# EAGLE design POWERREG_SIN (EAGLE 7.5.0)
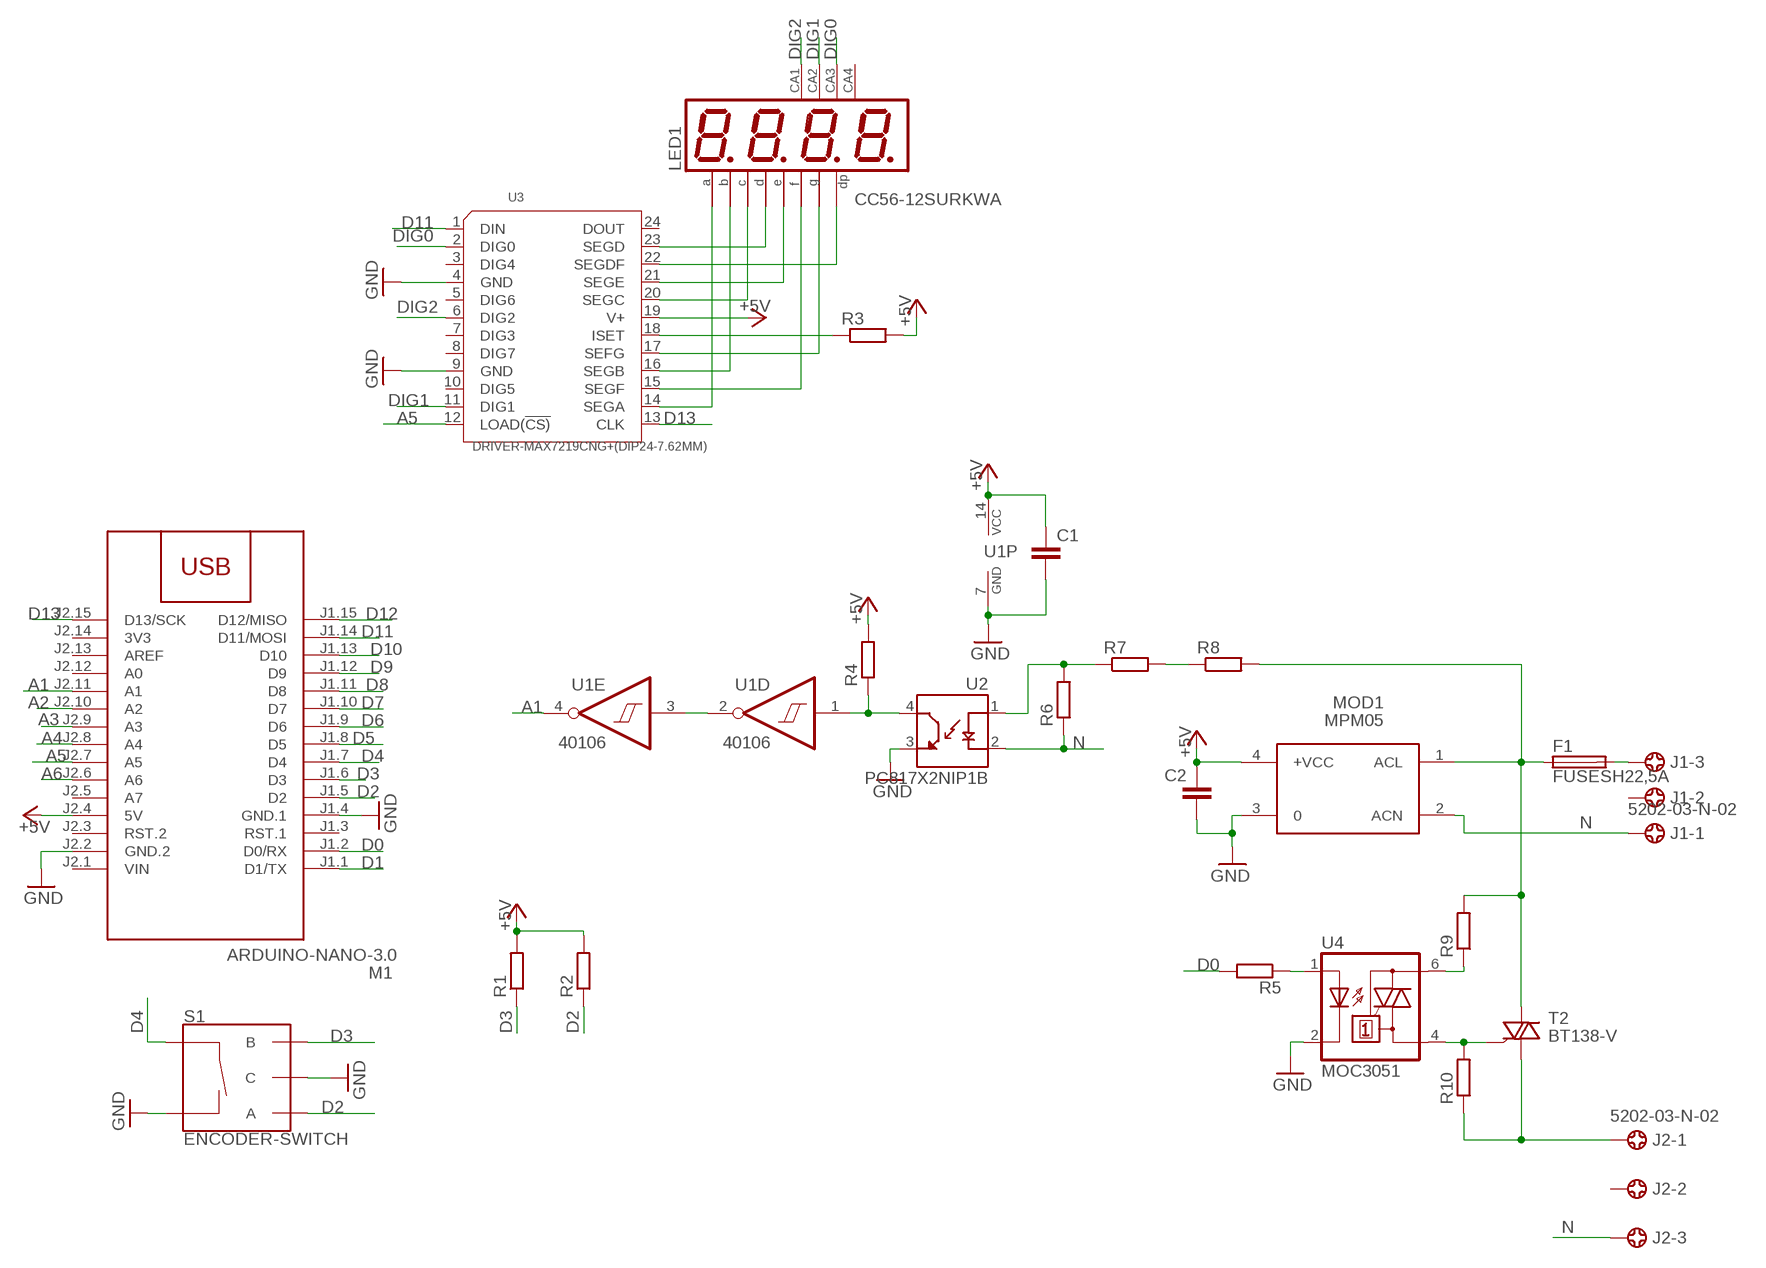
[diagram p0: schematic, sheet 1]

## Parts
C1  C-EUC1206  [C1206]
C2  C-EUC1206  [C1206]
F1  FUSESH22,5A  [SH22,5A]
J1  5202-03-N-02  [5202-03-N-02]
J2  5202-03-N-02  [5202-03-N-02]
LED1  CC56-12SURKWA  CA56-12SURKWA  [CA56-12SURKWA]
M1  ARDUINO-NANO-3.0  [ARDUINO-NANO-3.0]
MOD1  MPM05  [MPM05]
R1  R-EU_R1206  [R1206]
R2  R-EU_R1206  [R1206]
R3  R-EU_R1206  [R1206]
R4  R-EU_R1206  [R1206]
R5  R-EU_R1206  [R1206]
R6  R-EU_R2512  [R2512]
R7  R-EU_R2512  [R2512]
R8  R-EU_R2512  [R2512]
R9  R-EU_R1206  [R1206]
R10  R-EU_R1206  [R1206]
S1  ENCODER-SWITCH  [ROTARY_ENC_PLAIN]
T2  BT138-V  [TO220BV]
U1  40106  74HC14N  [DIL14]
U2  PC817X2NIP1B  [SOIC254P960X420-4N]
U3  DRIVER-MAX7219CNG+(DIP24-7.62MM)  [DIP24-2.54-30.6X7.62MM]
U4  MOC3051  MOC3042M  [DIL06]

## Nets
+5V: C1.1 C2.1 M1.J2.4(5V) MOD1.4(+VCC) R1.2 R2.2 R3.2 R4.2 U1.14(P:VCC) U3.19(V+)
A1: M1.J2.11(A1) U1.4(E:O)
A2: M1.J2.10(A2)
A3: M1.J2.9(A3)
A4: M1.J2.8(A4)
A5: M1.J2.7(A5) U3.12(LOAD(!CS))
A6: M1.J2.6(A6)
D0: M1.J1.2(D0/RX) R5.2
D1: M1.J1.1(D1/TX)
D2: M1.J1.5(D2) R2.1 S1.A
D3: M1.J1.6(D3) R1.1 S1.B
D4: M1.J1.7(D4) S1.SW+
D5: M1.J1.8(D5)
D6: M1.J1.9(D6)
D7: M1.J1.10(D7)
D8: M1.J1.11(D8)
D9: M1.J1.12(D9)
D10: M1.J1.13(D10)
D11: M1.J1.14(D11/MOSI) U3.1(DIN)
D12: M1.J1.15(D12/MISO)
D13: M1.J2.15(D13/SCK) U3.13(CLK)
DIG0: LED1.8(CA) U3.2(DIG0)
DIG1: LED1.9(CA) U3.11(DIG1)
DIG2: LED1.12(CA) U3.6(DIG2)
GND: C1.2 C2.2 M1.J1.4(GND.1) M1.J2.2(GND.2) MOD1.3 S1.C S1.SW- U1.7(P:GND) U2.3(ET) U3.4(GND) U3.9(GND) U4.2(C)
N: J1.1 J2.3 MOD1.2(ACN) R6.1 U2.2(C)
N$1: LED1.11(A) U3.14(SEGA)
N$2: LED1.10(F) U3.15(SEGF)
N$3: LED1.7(B) U3.16(SEGB)
N$4: LED1.5(G) U3.17(SEFG)
N$5: LED1.4(C) U3.20(SEGC)
N$6: LED1.2(D) U3.23(SEGD)
N$7: LED1.1(E) U3.21(SEGE)
N$8: LED1.3(DP) U3.22(SEGDF)
N$9: R3.1 U3.18(ISET)
N$10: F1.2 J1.3
N$11: F1.1 MOD1.1(ACL) R8.2 R9.2 T2.T2(A2)
N$12: R9.1 U4.6(A2)
N$13: R10.2 T2.G U4.4(A1)
N$14: J2.1 R10.1 T2.T1(A1)
N$15: R6.2 R7.1 U2.1(A)
N$16: R7.2 R8.1
N$17: R4.1 U1.1(D:I) U2.4(CT)
N$18: U1.2(D:O) U1.3(E:I)
N$19: R5.1 U4.1(A)
Unconnected: J1.2 J2.2 LED1.6(CA4) M1.J1.3(RST.1) M1.J2.3(RST.2) M1.J2.5(A7) M1.J2.12(A0) M1.J2.13(AREF) U1.5(F:I) U1.6(F:O) U1.8(C:O) U1.9(C:I) U1.10(B:O) U1.11(B:I) U1.12(A:O) U1.13(A:I) U3.3(DIG4) U3.5(DIG6) U3.7(DIG3) U3.8(DIG7) U3.10(DIG5) U3.24(DOUT)

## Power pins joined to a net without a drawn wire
3V3: M1.J2.14(3V3)
VIN: M1.J2.1(VIN)

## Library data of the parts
C1 C2 = rcl:C-EU: CAPACITOR, European symbol
F1 = fuse:FUSE: Fuse; OC_FARNELL: unknown; OC_NEWARK: unknown
J1 J2 = con-ebyelectro:5202-03-N-02: Barrier Blocks Sreies 5202 Source: http://www.ebyelectro.com/PDF/5202-XX-N-02.pdf; OC_FARNELL: unknown; OC_NEWARK: unknown
LED1 = display-kingbright:CA56-12SURKWA
M1 = diy-modules:ARDUINO-NANO-3.0: Arduino Nano 3.0 and compatible devices More details available here: https://www.arduino.cc/en/Main/ArduinoBoardNano Click here to find device on ebay.com
MOD1 = acdc:MPM05: AC DC Converter 5W
R1-R10 = rcl:R-EU_: RESISTOR, European symbol
S1 = SparkFun-Switches:ENCODER-SWITCH: Rotary Encoder w/ Select Switch Encoders rotate similarly to potentiometers, but they’re different from potentiometers in that an encoder has full rotation without limits. They output gray code so that you can tell how much and in which direction the encoder has been turned. This encoder includes a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; SF_SKU: COM-09117
T2 = triac:BT138: TRIAC Source: http://www.semiconductors.philips.com BT138_SERIES_2.pdf
U1 = 74xx-eu:74*14: Hex schmitt trigger INVERTER
U2 = PC817X2NIP1B:PC817X2NIP1B: Check availability; AVAILABILITY: In Stock; CHECK_PRICES: https://www.snapeda.com/parts/PC817X2NIP1B/Sharp/view-part/?ref=eda; DESCRIPTION: Optocoupler DC-IN 1-CH Transistor DC-OUT 4-Pin DIP SMD T/R; MF: Sharp Microelectronics; MP: PC817X2NIP1B; PACKAGE: SMD-4 Sharp Microelectronics; PRICE: None; SNAPEDA_LINK: https://www.snapeda.com/parts/PC817X2NIP1B/Sharp/view-part/?ref=snap
U3 = DRIVER-MAX7219CNG__DIP24-7.62MM_:DRIVER-MAX7219CNG+(DIP24-7.62MM): Check availability; AVAILABILITY: In Stock; CHECK_PRICES: https://www.snapeda.com/parts/MAX7219CNG+/Maxim+Integrated/view-part/?ref=eda; DESCRIPTION: LED Driver 64 Segment 330000uA Supply Current 24-Pin PDIP N Tube; MF: Maxim Integrated Products; MP: MAX7219CNG+; PACKAGE: PDIP-24 Maxim; PRICE: None; SNAPEDA_LINK: https://www.snapeda.com/parts/MAX7219CNG+/Maxim+Integrated/view-part/?ref=snap
U4 = optocoupler:MOC30*: 6-Pin DIP Zero-Cross Optoisolators Triac Driver Output (250/400 Volt Peak) Source: The old path of data sheet not more available 2013-05-06.; MF: FAIRCHILD SEMICONDUCTOR; MPN: MOC3042-M; OC_FARNELL: 1021368; OC_NEWARK: 72K8899

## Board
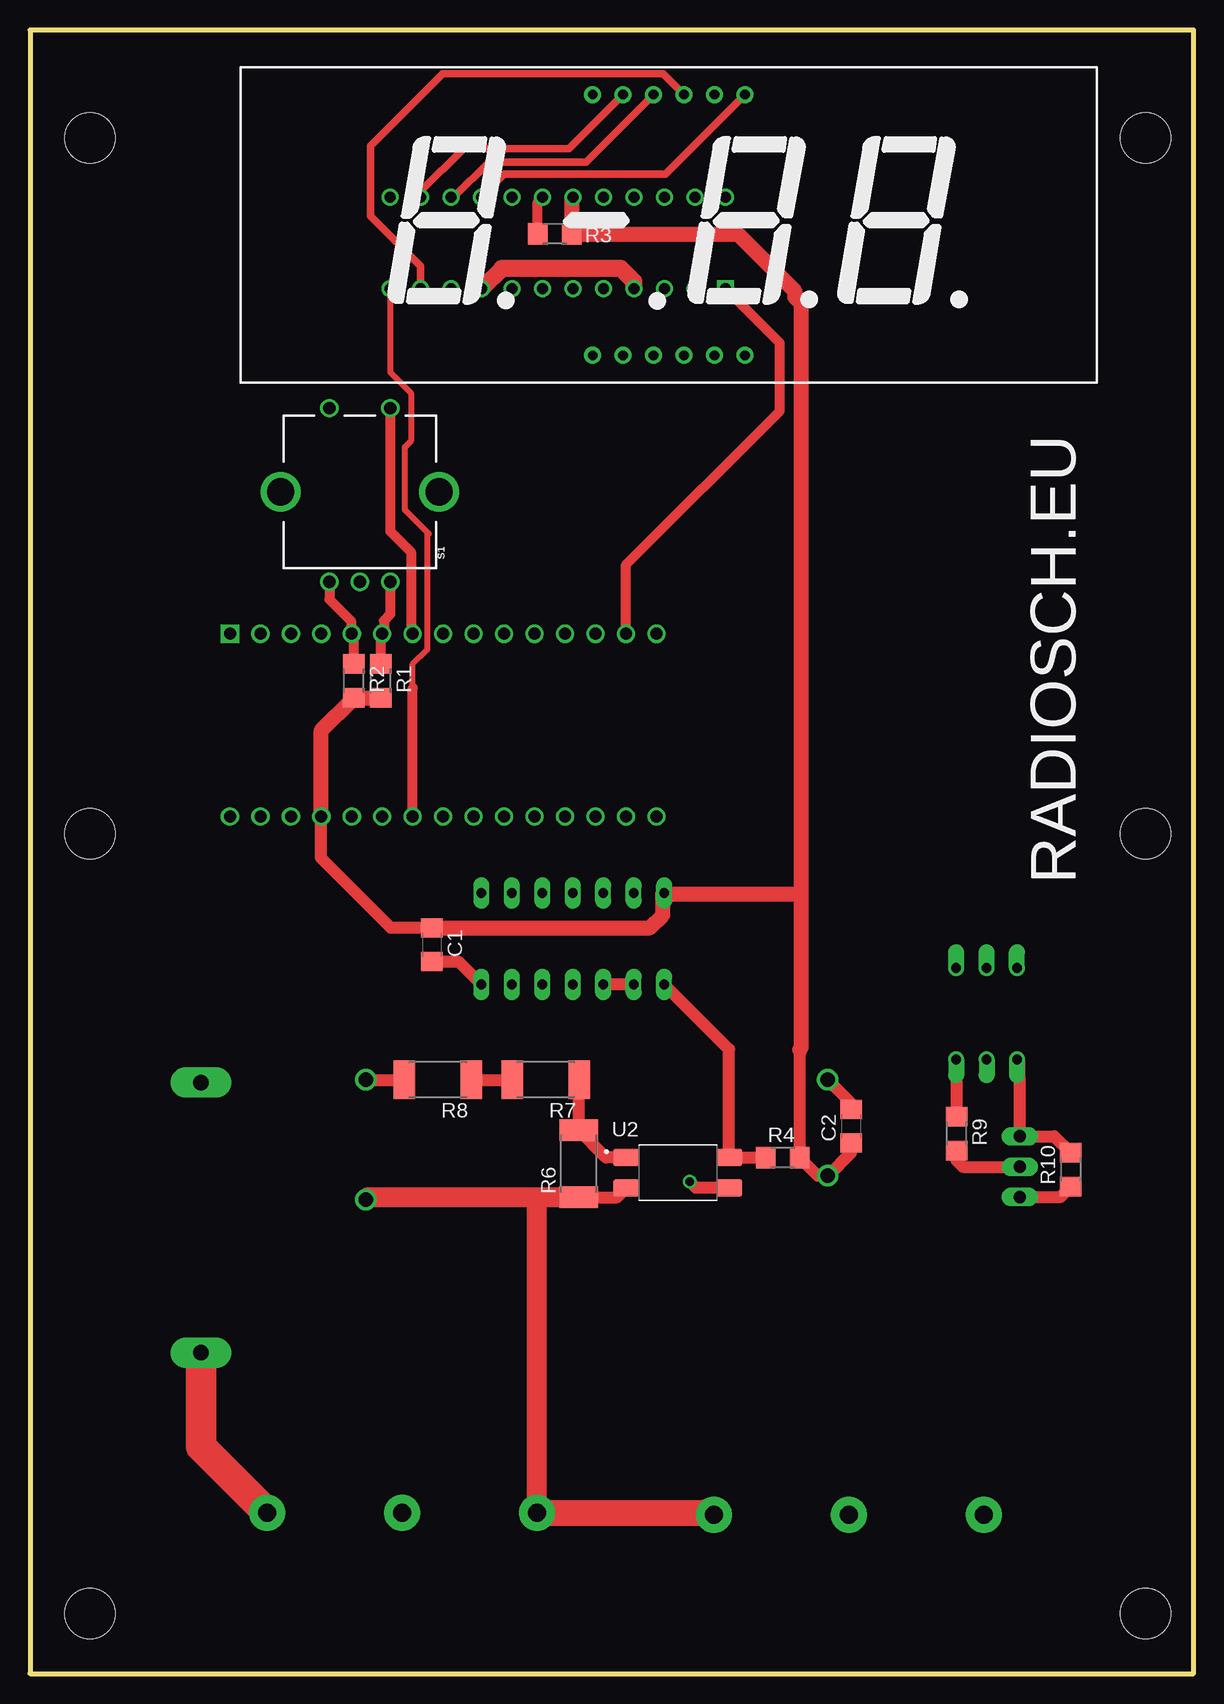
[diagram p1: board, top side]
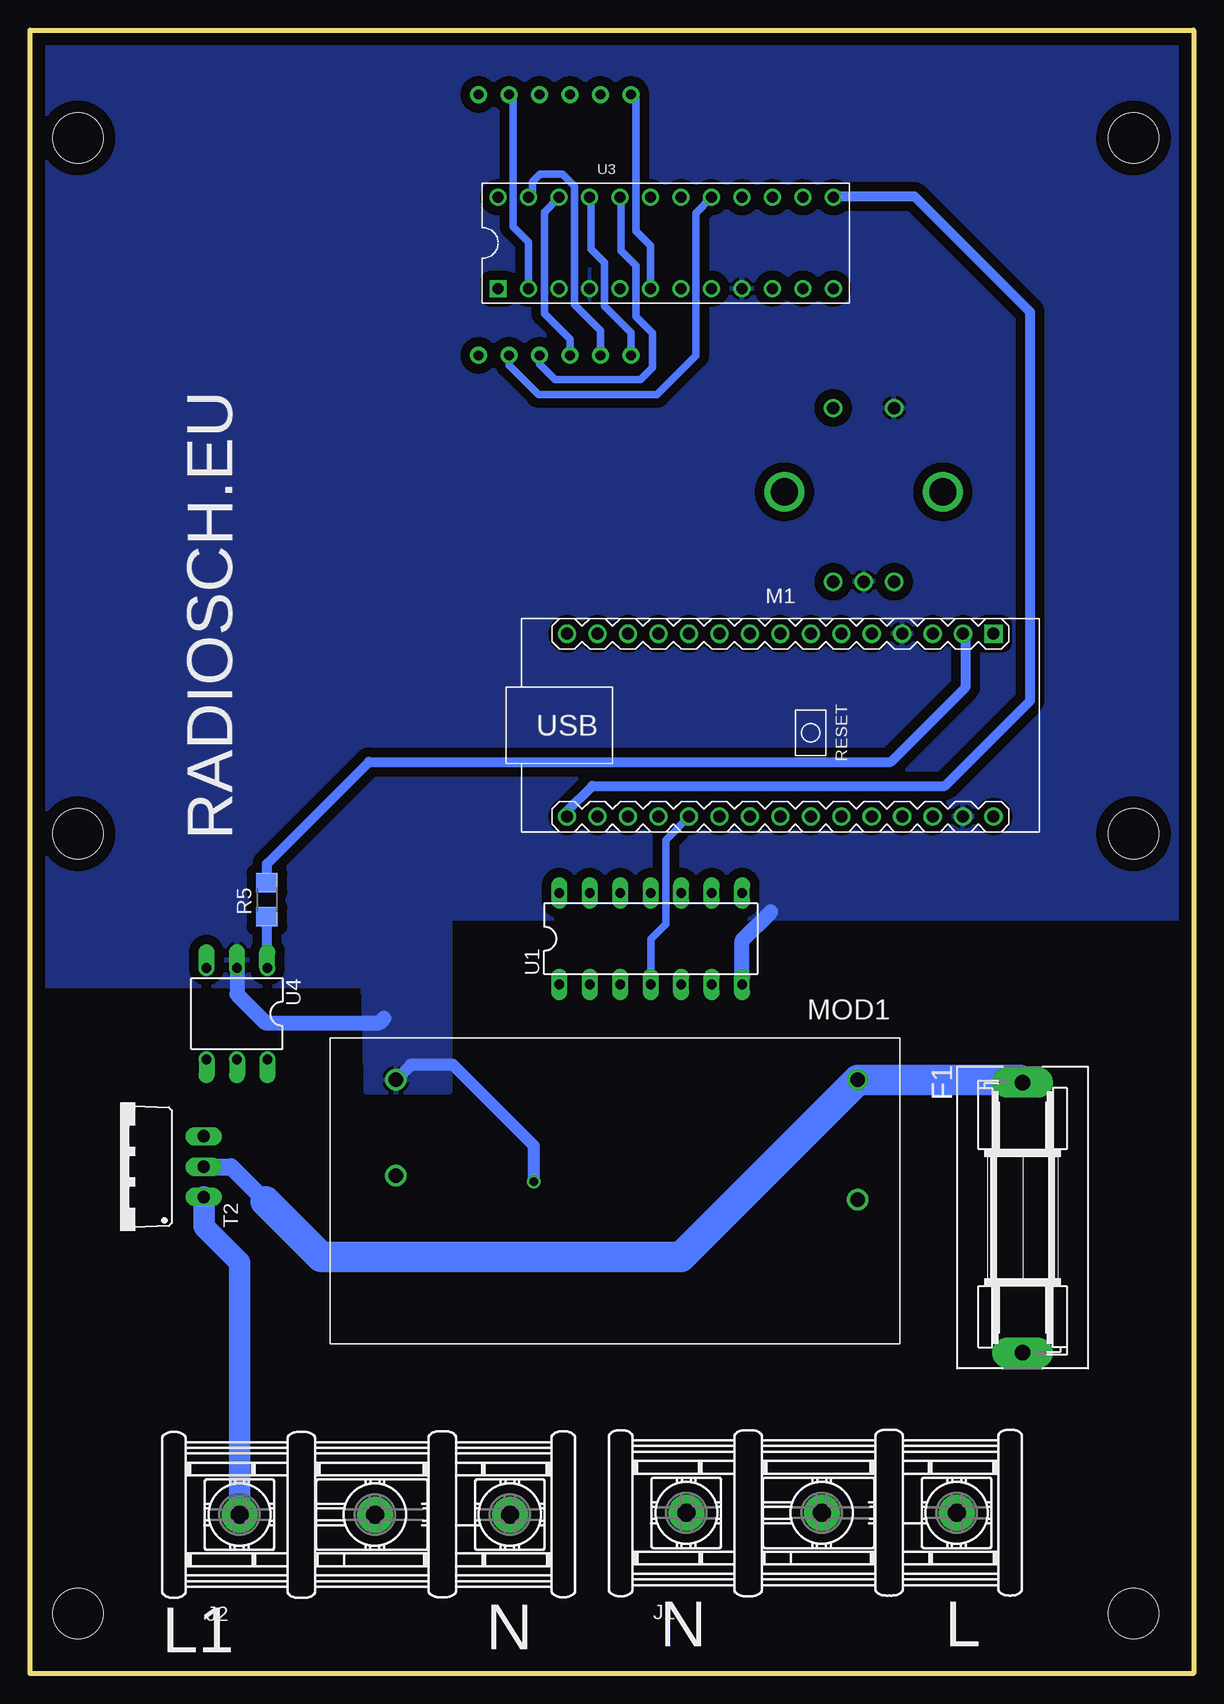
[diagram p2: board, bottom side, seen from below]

Size 97 x 137 mm. Coordinates in mm from the lower left corner, seen from the top.
Outline: 0,0 97,0 97,137 0,137 0,0
Copper layers (1*16): Top 0.035mm / dielectric 1.5mm / Bottom 0.035mm
Design rules "default": minimum track width 10mil, minimum drill 24mil, track to track 8mil, track to pad 8mil, pad to pad 8mil, via to via 8mil, smd to smd 8mil, copper to edge 40mil, drill to drill 8mil, minimum pad ring 10mil, minimum via ring 8mil, stop-mask expansion 4mil, vias tented up to drill 0mil, thermal gap 10mil
Holes 4.2 mm at 5,128 5,5 93,128 93,5 5,70 93,70

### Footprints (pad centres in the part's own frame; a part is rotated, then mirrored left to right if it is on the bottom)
C1206 = smd 1.6 x 1.8: 1 -1.4,0; 2 1.4,0
SH22,5A = drill 1.321 pad 2.54 long: 1 -11.252,0; 2 11.252,0
5202-03-N-02 = drill 1.5 pad 3: 1 -9.29,0; 2 2,0; 3 13.25,0
CA56-12SURKWA = drill 0.8 pad 1.422: 1 10.65,-7.12; 2 13.19,-7.12; 3 15.73,-7.12; 4 18.27,-7.12; 5 20.81,-7.12; 6 23.35,-7.12; 7 23.35,14.62; 8 20.81,14.62; 9 18.27,14.62; 10 15.73,14.62; 11 13.19,14.62; 12 10.65,14.62
ARDUINO-NANO-3.0 = drill 1 square: J1.1 17.78,7.62 | drill 1: J1.2 15.24,7.62; J1.3 12.7,7.62; J1.4 10.16,7.62; J1.5 7.62,7.62; J1.6 5.08,7.62; J1.7 2.54,7.62; J1.8 0,7.62; J1.9 -2.54,7.62; J1.10 -5.08,7.62; J1.11 -7.62,7.62; J1.12 -10.16,7.62; J1.13 -12.7,7.62; J1.14 -15.24,7.62; J1.15 -17.78,7.62; J2.1 17.78,-7.62; J2.2 15.24,-7.62; J2.3 12.7,-7.62; J2.4 10.16,-7.62; J2.5 7.62,-7.62; J2.6 5.08,-7.62; J2.7 2.54,-7.62; J2.8 0,-7.62; J2.9 -2.54,-7.62; J2.10 -5.08,-7.62; J2.11 -7.62,-7.62; J2.12 -10.16,-7.62; J2.13 -12.7,-7.62; J2.14 -15.24,-7.62; J2.15 -17.78,-7.62
MPM05 = drill 1.2: 1 3.5,-22; 2 3.5,-12; 3 42,-22; 4 42,-14
R1206 = smd 1.6 x 1.803: 1 -1.422,0; 2 1.422,0
R2512 = smd 1.8 x 3.2: 1 -2.8,0; 2 2.8,0
ROTARY_ENC_PLAIN = drill 1.016: A 7.493,-2.54; B 7.493,2.54; C 7.493,0; SW+ -6.985,2.54; SW- -6.985,-2.54 | drill 2.286: P$3 0,6.604; P$4 0,-6.604
TO220BV = drill 1.016 long: G 2.54,-6.985; T1 -2.54,-6.985; T2 0,-6.985
DIL14 = drill 0.813 long: 1 -7.62,-3.81; 2 -5.08,-3.81; 3 -2.54,-3.81; 4 0,-3.81; 5 2.54,-3.81; 6 5.08,-3.81; 7 7.62,-3.81; 8 7.62,3.81; 9 5.08,3.81; 10 2.54,3.81; 11 0,3.81; 12 -2.54,3.81; 13 -5.08,3.81; 14 -7.62,3.81
SOIC254P960X420-4N = smd 2.15 x 1.48: 1 -4.28,1.27; 2 -4.28,-1.27; 3 4.28,-1.27; 4 4.28,1.27
DIP24-2.54-30.6X7.62MM = drill 0.9 pad 1.4 square: 1 -13.97,-3.81 | drill 0.9 pad 1.4: 2 -11.43,-3.81; 3 -8.89,-3.81; 4 -6.35,-3.81; 5 -3.81,-3.81; 6 -1.27,-3.81; 7 1.27,-3.81; 8 3.81,-3.81; 9 6.35,-3.81; 10 8.89,-3.81; 11 11.43,-3.81; 12 13.97,-3.81; 13 13.97,3.81; 14 11.43,3.81; 15 8.89,3.81; 16 6.35,3.81; 17 3.81,3.81; 18 1.27,3.81; 19 -1.27,3.81; 20 -3.81,3.81; 21 -6.35,3.81; 22 -8.89,3.81; 23 -11.43,3.81; 24 -13.97,3.81
DIL06 = drill 0.813 offset: 1 -2.54,-3.81; 2 0,-3.81; 3 2.54,-3.81; 4 2.54,3.81; 5 0,3.81; 6 -2.54,3.81

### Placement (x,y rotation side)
C1  33.5,60.75 270 top
C2  68.47,45.62 90 top
F1  14.25,38 270 bottom
J1  33,13.39 0 bottom
J2  70.25,13.25 0 bottom
LED1  36.25,117 0 top
M1  34.45,79.05 0 bottom
MOD1  24.5,27.5 180 bottom
R1  29.25,82.75 270 top
R2  27,82.75 270 top
R3  43.75,120 0 top
R4  62.75,43 0 top
R5  77.25,64.5 90 bottom
R6  45.75,42.5 90 top
R7  43,49.5 180 top
R8  34,49.5 180 top
R9  77.25,45 270 top
R10  86.75,42 90 top
S1  27.5,98.5 270 top
T2  89.5,42.25 90 bottom
U1  45.25,61.25 0 bottom
U2  54,41.75 0 top
U3  44,119.25 0 bottom
U4  79.75,55 180 bottom

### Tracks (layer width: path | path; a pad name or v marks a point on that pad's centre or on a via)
+5V
  Top 1.016: 64.17,53.76 64.17,52 R4.2 65.67,41.5 MOD1.4 68.47,43.47 C2.1 | C1.1 30.1,62.15 24.25,68 24.25,71.39 M1.J2.4
  Top 1.27: 64.25,65 64.25,114.25 63.75,114.75 63.75,115.25 59,120 R3.2 45.17,122.96 U3.19 | 64.25,65 64.25,52.08 64.17,52 | C1.1 51.65,62.15 52.75,63.25 52.75,64.94 | 52.75,64.94 U1.14 | 52.75,64.94 52.75,65 64.25,65 | M1.J2.4 24.29,78.62 R2.2 R1.2
A1
  Bottom 0.61: U1.4 45.25,61.25 44,62.5 44,69.5 M1.J2.11
A5
  Top 0.5: 33.25,95 33.12,95.12 | 33.12,95.12 31.25,97 31.25,102.25 31.75,102.75 31.75,106.75 30.03,108.47 U3.12 | 31.91,82.16 31.91,84.16 33.12,85.38 33.12,95.12
  Top 0.813: M1.J2.7 31.91,82.16
D0
  Bottom 0.813: R5.2 77.25,67.5 68.75,76 25.25,76 19,82.25 19,86.46 M1.J1.2
D2
  Top 0.813: S1.A 24.96,89.54 26.75,87.75 26.75,86.75 M1.J1.5 27,86.5 R2.1
D3
  Top 0.813: S1.B 30.04,88.29 29.5,87.75 29.5,86.8 M1.J1.6 29.25,86.55 R1.1
D4
  Top 0.813: S1.SW+ 30.04,95.21 31.75,93.5 31.75,86.83 M1.J1.7
D11
  Top 0.813: M1.J1.14 49.69,92.44 62.5,105.25 62.5,110.91 U3.1
D13
  Bottom 0.813: M1.J2.15 52.23,71.9 50.12,74 20.75,74 13.62,81.12 13.62,113.5 23.25,123.12 29.96,123.12 U3.13
DIG0
  Bottom 0.61: U3.2 55.43,119.31 56.75,120.62 56.75,131.31 LED1.8
DIG1
  Top 0.61: U3.11 32.57,117.31 28.38,121.5 28.38,127.38 34.38,133.38 52.77,133.38 LED1.9
DIG2
  Bottom 0.61: U3.6 45.27,119.02 46.5,120.25 46.5,131.22 LED1.12
GND  (via drill 0.7)
  Top 1.016: C2.2 68.47,47.53 MOD1.3 | U2.3 55.52,40.48 v55,41 | C1.2 35.72,59.35 U1.7
  Top 1.422: U3.4 50.35,116.03 49.25,117.12 39.34,117.12 U3.9
  Bottom 1.016: v55,41 55,44 61.75,50.75 65.25,50.75 MOD1.3
  Bottom 1.27: U1.7 37.63,61.12 35.25,63.5 | U4.2 79.75,56.62 77.38,54.25 67.88,54.25 67.5,54.62
  pour Bottom (isolate 0.8): 1,137 96,137 96.25,57.38 69.25,57.38 69,48.5 62,48.5 62,63 1,63
N
  Top 1.016: R6.1 48.94,39.7 U2.2
  Top 1.676: R6.1 42.5,39.7 | 42.5,39.7 28.2,39.7 MOD1.2 | J1.1 42.29,39.49 42.5,39.7
  Top 2.184: J1.1 56.39,13.39 56.5,13.5 56.75,13.5 J2.3
N$1
  Top 0.61: U3.14 32.57,123.57 36.12,127.12 44.95,127.12 LED1.11
N$2
  Top 0.61: U3.15 35.31,123.06 38.25,126 46.36,126 LED1.10
N$3
  Top 0.61: U3.16 37.65,123.15 39.5,125 52.98,125 LED1.7
N$4
  Bottom 0.61: LED1.5 57.06,109.06 54.62,106.62 44.75,106.62 41.5,109.88 41.5,121.75 U3.17
N$5
  Bottom 0.61: LED1.4 54.52,109.14 53.25,107.88 46.12,107.88 45.12,108.88 45.12,111.75 46.5,113.12 46.5,117.38 47.75,118.62 47.75,123 U3.20
N$6
  Bottom 0.61: LED1.2 49.44,111.94 51.62,114.12 51.62,124 52.62,125 54.5,125 55.12,124.38 55.12,123.36 U3.23
N$7
  Bottom 0.61: LED1.1 46.9,111.78 49.12,114 49.12,117.62 50.25,118.75 50.25,122.96 U3.21
N$8
  Bottom 0.61: LED1.3 51.98,111.23 54.12,113.38 54.12,121.83 U3.22
N$9
  Top 0.813: R3.1 42.33,122.66 U3.18
N$10
  Top 2.54: F1.2 14.25,18.89 J1.3
N$11
  Top 1.016: MOD1.1 R8.2 | R9.2 77.25,42.75 77.75,42.25 T2.T2
  Bottom 1.27: 14.5,49.5 F1.1
  Bottom 1.422: T2.T2 80.25,42.25 77.38,39.38 77,39
  Bottom 2.54: 77.38,39.38 72.75,34.75 42.75,34.75 MOD1.1 14.5,49.5
N$12
  Top 1.016: R9.1 77.25,51.15 U4.6
N$13
  Top 1.016: R10.2 85.38,44.79 T2.G 82.52,50.97 U4.4
N$14
  Top 1.016: T2.T1 85.88,39.71 R10.1
  Bottom 1.778: J2.1 79.54,34.29 82.5,37.25 82.5,39.7 T2.T1
N$15
  Top 1.016: R7.1 45.75,49.45 R6.2 48.03,43.02 U2.1
N$16
  Top 1.016: R8.1 R7.2
N$17
  Top 1.016: R4.1 61.31,43.02 U2.4 58.28,52.03 U1.1
N$18
  Top 1.016: U1.2 U1.3
N$19
  Bottom 0.813: U4.1 77.21,63.04 R5.1

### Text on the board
tPlace: RADIOSCH.EU
bPlace: RADIOSCH.EU | L | N | N | L1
